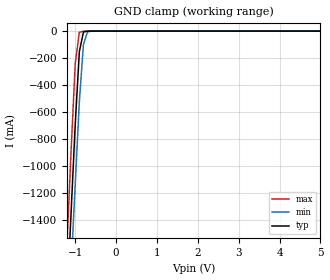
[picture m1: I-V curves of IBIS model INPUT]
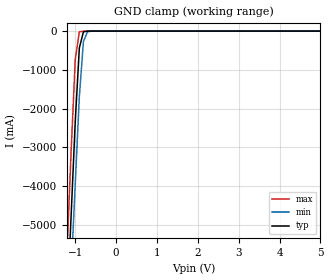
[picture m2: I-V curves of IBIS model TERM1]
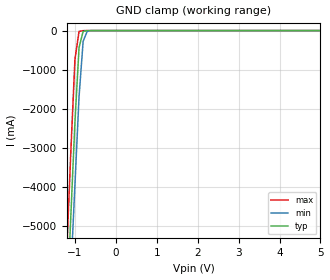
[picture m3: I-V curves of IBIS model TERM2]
|   PERICOM SEMICONDUCTOR CORP
|   IBIS Model of PI5C3126
|   Product Family: 5C
|   TSSOP (L) Package
[IBIS Ver] 3.2
[Comment char] |_char
[File Name] pi5c3126_l_50v.ibs
[File Rev] 1.0
[Source] File originated at Pericom Semiconductor Corp.
[Date] 05/09/14
[Disclaimer] (C) Copyright PERICOM Semiconductor Corporation
   All rights reserved
  Pericom Semiconductor Corporation hereby grants the user of
  this IBIS model a non-exclusive, nontransferable license to
  use this IBIS model under the following terms.
  This IBIS model is provided on an "AS IS" basis and Pericom
  makes absolutely no warranty with respect to the information
  contained herein. PERICOM DISCLAIMS AND CUSTOMER WAIVES ALL
  WARRANTIES, EXPRESSED OR IMPLIED, INCLUDING WARRANTIES OF
  MERCHANTABILITY OR FITNESS FOR A PARTICULAR PURPOSE. The
  entire risk as to quality and performance is with the customer.
  Accordingly, in no event shall the company be liable for any
  damages, whether in contract or tort, including any lost
  profits or other incidental, consequential, exemplary, or
  punitive damages arising out of the use or application of the
  IBIS model provided in this package. Further, Pericom reserves
  the right to make changes without notice to any product herein
  to improve reliability, function, or design. Pericom does not
  convey any license under patent rights or any other intellectual
  property rights, including those of third parties.
  The user is granted this license only to use the IBIS model
  and is not granted rights to sell, load, rent, lease or license
  the IBIS model in whole or in part, or in modified form to anyone
  other than user. User may modify the IBIS model to suit its specific
  application but rights to derivative works and such modifications
  shall belong to Pericom.
  Pericom is not obligated to provide maintenance or support
  for the licensed IBIS model.
  Contact Pericom at ATTN: APPLICATION ENGINEERING / IBIS MODELS
  1545 Barber Lane Milpitas, CA 95035 USA.
[Component] PI5C3126
[Manufacturer] Pericom Semiconductor Corp.
[Package]
| variable   typ   min   max
R_pkg   0.05665ohm   0.05334ohm   0.05997ohm
L_pkg   2.44150nH   2.12200nH   2.76100nH
C_pkg   0.20800pF   0.16300pF   0.25300pF
[Pin] signal_name   model_name   R_pin   L_pin   C_pin
1   BE0   INPUT   0.05997   2.76100nH   0.25300pF
2   A0   TERM1   0.05776   2.54800nH   0.22300pF
3   B0   TERM2   0.05555   2.33500nH   0.19300pF
4   BE1   INPUT   0.05334   2.12200nH   0.16300pF
5   A1   TERM1   0.05555   2.33500nH   0.19300pF
6   B1   TERM2   0.05776   2.54800nH   0.22300pF
7   GND   GND   0.05997   2.76100nH   0.25300pF
8   B2   TERM2   0.05997   2.76100nH   0.25300pF
9   A2   TERM1   0.05776   2.54800nH   0.22300pF
10   BE2   INPUT   0.05555   2.33500nH   0.19300pF
11   B3   TERM2   0.05334   2.12200nH   0.16300pF
12   A3   TERM1   0.05555   2.33500nH   0.19300pF
13   BE3   INPUT   0.05776   2.54800nH   0.22300pF
14   VCC   POWER   0.05997   2.76100nH   0.25300pF
[Series Switch Groups]
On 1 /
[Series_Pin_Mapping]   pin_2   model_name   function_table_group
2   3   SWITCH1   1
5   6   SWITCH1   1
9   8   SWITCH1   1
12   11   SWITCH1   1
|   Model SWITCH1
[Model] SWITCH1
Model_type Series_switch
| variable   typ   min   max
C_comp   8.0000pF   7.9200pF   8.0800pF
[Voltage Range]   5.0000V   4.5000V   5.5000V
[temperature range]   25   85   -40
[On]
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[OFF]
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| Models and submodels in the file (4): INPUT (Input), SWITCH1 (Series_switch), TERM1 (Terminator), TERM2 (Terminator)
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|   Model INPUT
[Model] INPUT
Model_type Input
Vinl = 1.500V
Vinh = 3.500V
| variable   typ   min   max
C_comp   6.0000pF   5.9400pF   6.0600pF
[Voltage Range]   5.0000V   4.5000V   5.5000V
[temperature range]   25   85   -40
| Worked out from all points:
|   GND clamp passes 1 mA (typ) near -0.71 V on its own axis
[GND Clamp]
| Voltage   I(typ)   I(min)   I(max)
-5V       -26.43A    -25.51A    -27.59A
-1.2V     -1.976A    -2.351A    -1.561A
-1.1V     -1.333A    -1.742A    -876.1mA
-1V       -689.5mA   -1.133A    -237.7mA
-900mV    -152.8mA   -525.5mA   -8.619mA
-800mV    -7.512mA   -99.97mA   -842.8uA
-700mV    -518.9uA   -6.478mA   -104.3uA
-500mV    -3.741uA   -32.95uA   -179.2nA
5V        81.04pA    180.4pA    80.01pA
[POWER Clamp]
| Voltage   I(typ)   I(min)   I(max)
-5V       0A         0A         0A
0V        0A         0A         0A
|   Model TERM1
[Model] TERM1
Model_type Terminator
| variable   typ   min   max
C_comp   6.0000pF   5.9400pF   6.0600pF
[Voltage Range]   5.0000V   4.5000V   5.5000V
[temperature range]   25   85   -40
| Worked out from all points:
|   GND clamp passes 1 mA (typ) near -0.69 V on its own axis
[GND Clamp]
| Voltage   I(typ)   I(min)   I(max)
-5V       -98.4A     -94.6A     -103.2A
-1.2V     -7.136A    -8.475A    -5.649A
-1.1V     -4.734A    -6.209A    -3.081A
-1V       -2.333A    -3.943A    -732.6mA
-900mV    -436.8mA   -1.694A    -20.9mA
-800mV    -19.19mA   -272.2mA   -1.375mA
-700mV    -1.088mA   -17.12mA   -157.3uA
-500mV    -5.777uA   -75.55uA   -268.9nA
5V        184pA      267.6pA    183.2pA
[POWER Clamp]
| Voltage   I(typ)   I(min)   I(max)
-5V       0A         0A         0A
0V        0A         0A         0A
|   Model TERM2
[Model] TERM2
Model_type Terminator
| variable   typ   min   max
C_comp   6.0000pF   5.9400pF   6.0600pF
[Voltage Range]   5.0000V   4.5000V   5.5000V
[temperature range]   25   85   -40
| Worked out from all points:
|   GND clamp passes 1 mA (typ) near -0.69 V on its own axis
[GND Clamp]
| Voltage   I(typ)   I(min)  I(max)
-5V       -98.4A     -94.6A     -103.2A
-1.2V     -7.136A    -8.475A    -5.649A
-1.1V     -4.734A    -6.209A    -3.081A
-1V       -2.333A    -3.943A    -732.6mA
-900mV    -436.8mA   -1.694A    -20.9mA
-800mV    -19.19mA   -272.2mA   -1.375mA
-700mV    -1.088mA   -17.12mA   -157.3uA
-500mV    -5.777uA   -75.55uA   -268.9nA
5V        184pA      267.5pA    183.2pA
[POWER Clamp]
| Voltage   I(typ)   I(min)   I(max)
-5V       0A         0A         0A
0V        0A         0A         0A
